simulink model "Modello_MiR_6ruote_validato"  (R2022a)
settings: Solver=VariableStepAuto  StartTime=0.0  StopTime=time_s(end,1)  RelTol=1e-3
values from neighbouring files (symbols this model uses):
  a = 0.250    (= 0.25)    [Modello_MiR_6ruote_validato_script.m]    (also in Modello_MiR_2ruote_script.m; Modello_MiR_6ruote_script.m; Modello_MiR_UR_script.m)
  a1 = 0.18265    [Modello_MiR_6ruote_validato_script.m]    (also in Modello_MiR_2ruote_script.m = deg2rad(5); Modello_MiR_6ruote_script.m = deg2rad(5); Modello_MiR_UR_script.m; UR_DHtable_e.m = 0)
  a2 = 0.40857    [Modello_MiR_6ruote_validato_script.m]    (also in Modello_MiR_2ruote_script.m = deg2rad(25); Modello_MiR_6ruote_script.m = deg2rad(25); Modello_MiR_UR_script.m; UR_DHtable_e.m = 612)
  Att_C1 = 0.01    [Modello_MiR_6ruote_validato_script.m]    (also in Modello_MiR_UR_script.m)
  Att_C2 = 0.01    [Modello_MiR_6ruote_validato_script.m]    (also in Modello_MiR_UR_script.m)
  Att_C5 = 0.01    [Modello_MiR_6ruote_validato_script.m]    (also in Modello_MiR_UR_script.m)
  Att_C6 = 0.01    [Modello_MiR_6ruote_validato_script.m]    (also in Modello_MiR_UR_script.m)
  b = 0.1875    [Modello_MiR_6ruote_validato_script.m]    (also in Modello_MiR_2ruote_script.m; Modello_MiR_6ruote_script.m; Modello_MiR_UR_script.m)
  b_caster = 0.07    [Modello_MiR_6ruote_validato_script.m]    (also in Modello_MiR_2ruote_script.m; Modello_MiR_6ruote_script.m; Modello_MiR_UR_script.m)
  bd = 0.205    [Modello_MiR_6ruote_validato_script.m]    (also in Modello_MiR_2ruote_script.m; Modello_MiR_6ruote_script.m; Modello_MiR_UR_script.m)
  F23fun = @(u) (mv*9.801/4)-(mv*h*u(5)+(mv*9.801/4)*(2*a-b_caster*(cos(u(1))+cos(u(2)))))/(4*a-b_caster*(cos(u(1))+cos(u(2)))+b_caster*(cos(u(3))+cos(u(4))))    [Modello_MiR_6ruote_validato_script.m]    (also in Modello_MiR_6ruote_script.m = @(u) (mv*9.801/4)-u(7))
  F43fun = @(u) (1/(2*bd))*(mv*u(6)*h+((mv*h*u(5)+(mv*9.801/4)*(2*a-b_caster*(cos(u(1))+cos(u(2)))))/(4*a-b_caster*(cos(u(1))+cos(u(2)))+b_caster*(cos(u(3))+cos(u(4)))))*(2*bd-b_caster*(sin(u(3))+sin(u(4))))+((mv*9.801/4)-(mv*h*u(5)+(mv*9.801/4)*(2*a-b_caster*(cos(u(1))+cos(u(2)))))/(4*a-b_caster*(cos(u(1))+cos(u(2)))+b_caster*(cos(u(3))+cos(u(4)))))*(2*bd-b_caster*(sin(u(1))+sin(u(2)))))    [Modello_MiR_6ruote_validato_script.m]    (also in Modello_MiR_6ruote_script.m = @(u) (1/(2*bd))*(mv*u(6)*h+u(7)*(2*bd-b_caster*(sin(u(3))+si)
  F63fun = @(u) (mv*h*u(5)+(mv*9.801/4)*(2*a-b_caster*(cos(u(1))+cos(u(2)))))/(4*a-b_caster*(cos(u(1))+cos(u(2)))+b_caster*(cos(u(3))+cos(u(4))))    [Modello_MiR_6ruote_validato_script.m]    (also in Modello_MiR_6ruote_script.m)
  f_c = 0.29564    [Modello_MiR_6ruote_validato_script.m]    (also in Modello_MiR_UR_script.m)
  f_d3 = 0.35846    [Modello_MiR_6ruote_validato_script.m]    (also in Modello_MiR_UR_script.m)
  f_d4 = 0.2333    [Modello_MiR_6ruote_validato_script.m]    (also in Modello_MiR_UR_script.m)
  fa_c = 0.27474    [Modello_MiR_6ruote_validato_script.m]    (also in Modello_MiR_UR_script.m)
  fa_d3 = 0.3694    [Modello_MiR_6ruote_validato_script.m]    (also in Modello_MiR_UR_script.m)
  fa_d4 = 0.28065    [Modello_MiR_6ruote_validato_script.m]    (also in Modello_MiR_UR_script.m)
  fm_fun = @(u) (u <= -am2 || u >= am2) * 0 + (u > -am2 && u <= -am1) * (- u* Mza/(am2 -am1) - Mza* am2/(am2 -am1)) +           + (u > -am1 && u <= am1) * (Mza * u / am1) + (u > am1 && u < am2) * (Mza * u /(am1 -am2) - Mza * am2 /(am1 - am2))    [Modello_MiR_6ruote_validato_script.m]    (also in Modello_MiR_6ruote_script.m = @(u) (u <= -am2 | u >= am2)*0 + (u > -am2 && u <= -am1)*(- u; Modello_MiR_UR_script.m)
  Icw_1 = 1/2 * mcw * rc^2    (= 0.002004225735)    [Modello_MiR_6ruote_validato_script.m]    (also in Modello_MiR_2ruote_script.m; Modello_MiR_6ruote_script.m; Modello_MiR_UR_script.m)
  Icw_2 = 1/12 * mcw * ec^2 + 1/4 * mcw * rc^2    (= 0.00104098243873)    [Modello_MiR_6ruote_validato_script.m]    (also in Modello_MiR_2ruote_script.m; Modello_MiR_6ruote_script.m; Modello_MiR_UR_script.m)
  Idw_1 = 1/2 * mdw * rd^2    (= 0.00551836278784)    [Modello_MiR_6ruote_validato_script.m]    (also in Modello_MiR_2ruote_script.m; Transfer_Function_Gol_Gcl.m = Inertia_vect(jj,1); Modello_MiR_6ruote_script.m; Modello_MiR_UR_script.m)
  iMax = 20.7*1.1    (= 22.77)    [Modello_MiR_6ruote_validato_script.m]    (also in Modello_MiR_2ruote_script.m; Modello_MiR_6ruote_script.m; Modello_MiR_UR_script.m)
  Iv = mv * (l^2 + w^2)  / 12    (= 8.95033333333)    [Modello_MiR_6ruote_validato_script.m]    (also in Modello_MiR_2ruote_script.m = 6.75343333333; Modello_MiR_6ruote_script.m = 6.75343333333; Modello_MiR_UR_script.m = 6.75343333333)
  Kc = 0.15    [Modello_MiR_6ruote_validato_script.m]    (also in Modello_MiR_2ruote_script.m; Modello_MiR_6ruote_script.m; Modello_MiR_UR_script.m)
  Ki_i = 1    [Modello_MiR_6ruote_validato_script.m]    (also in Modello_MiR_2ruote_script.m; Modello_MiR_6ruote_script.m; Modello_MiR_UR_script.m)
  Ki_v = 1    [Modello_MiR_6ruote_validato_script.m]    (also in Modello_MiR_2ruote_script.m; Modello_MiR_6ruote_script.m; Modello_MiR_UR_script.m)
  kk = 0.00005    (= 5e-05)    [Modello_MiR_6ruote_validato_script.m]    (also in Modello_MiR_2ruote_script.m; Modello_MiR_6ruote_script.m; Modello_MiR_UR_script.m)
  Kp_i = 5    [Modello_MiR_6ruote_validato_script.m]    (also in Modello_MiR_2ruote_script.m; Modello_MiR_6ruote_script.m; Modello_MiR_UR_script.m)
  Kp_v = 5    [Modello_MiR_6ruote_validato_script.m]    (also in Modello_MiR_2ruote_script.m; Modello_MiR_6ruote_script.m; Modello_MiR_UR_script.m)
  kv = 1.5e-6    (= 1.5e-06)    [Modello_MiR_6ruote_validato_script.m]    (also in Modello_MiR_2ruote_script.m; Modello_MiR_6ruote_script.m; Modello_MiR_UR_script.m)
  L = R * tauE    (= 0.00181134822805)    [Modello_MiR_6ruote_validato_script.m]    (also in Modello_MiR_2ruote_script.m; Modello_MiR_6ruote_script.m; Modello_MiR_UR_script.m)
  mcw = rc^2 * pi * ec * rhopoliu + 1    (= 1.02616357632)    [Modello_MiR_6ruote_validato_script.m]    (also in Modello_MiR_2ruote_script.m; Modello_MiR_6ruote_script.m; Modello_MiR_UR_script.m)
  mv = 110    [Modello_MiR_6ruote_validato_script.m]    (also in Modello_MiR_2ruote_script.m = 83; Modello_MiR_6ruote_script.m = 83; Modello_MiR_UR_script.m = 83)
  Phi1_start = psi_mir(1,1)    [Modello_MiR_6ruote_validato_script.m]    (also in Modello_MiR_UR_script.m)
  Phi2_start = psi_mir(1,1)    [Modello_MiR_6ruote_validato_script.m]    (also in Modello_MiR_UR_script.m)
  Phi5_start = psi_mir(1,1)    [Modello_MiR_6ruote_validato_script.m]    (also in Modello_MiR_UR_script.m)
  Phi6_start = psi_mir(1,1)    [Modello_MiR_6ruote_validato_script.m]    (also in Modello_MiR_UR_script.m)
  Psi_start = psi_mir(1,1)    [Modello_MiR_6ruote_validato_script.m]    (also in Modello_MiR_6ruote_script.m = 1.57079632679; Modello_MiR_UR_script.m)
  R = velMax * TorqueMax / (iMax)^2    (= 1.81134822805)    [Modello_MiR_6ruote_validato_script.m]    (also in Modello_MiR_2ruote_script.m; Modello_MiR_6ruote_script.m; Modello_MiR_UR_script.m)
  rap_rid = 10.167    [Modello_MiR_6ruote_validato_script.m]    (also in Modello_MiR_2ruote_script.m; Modello_MiR_6ruote_script.m; Modello_MiR_UR_script.m)
  rc = 0.125/2    (= 0.0625)    [Modello_MiR_6ruote_validato_script.m]    (also in Modello_MiR_2ruote_script.m; Modello_MiR_6ruote_script.m; Modello_MiR_UR_script.m)
  rd = 0.1    [Modello_MiR_6ruote_validato_script.m]    (also in Modello_MiR_2ruote_script.m; Modello_MiR_6ruote_script.m; Modello_MiR_UR_script.m)
  s1 = 0.18987    [Modello_MiR_6ruote_validato_script.m]    (also in Modello_MiR_2ruote_script.m = 0.2; Modello_MiR_6ruote_script.m = 0.2; Modello_MiR_UR_script.m)
  s2 = 0.99533    [Modello_MiR_6ruote_validato_script.m]    (also in Modello_MiR_2ruote_script.m = 0.8; Modello_MiR_6ruote_script.m = 0.8; Modello_MiR_UR_script.m)
  Sx = spline(x ,fl_fun(x),zx)    [Modello_MiR_6ruote_script.m]
  Sy = spline(x ,ft_fun(x),zy)    [Modello_MiR_6ruote_script.m]
  VaMax = Kc * velMax    (= 41.2443991527)    [Modello_MiR_6ruote_validato_script.m]    (also in Modello_MiR_2ruote_script.m; Modello_MiR_6ruote_script.m; Modello_MiR_UR_script.m)
  X_start = traj(1,1)    [Modello_MiR_6ruote_validato_script.m]    (also in Modello_MiR_2ruote_script.m = input('Inserire coordinata x iniziale'); Modello_MiR_6ruote_script.m = input('Inserire coordinata x iniziale'); Modello_MiR_UR_script.m)
  Y_start = traj(1,2)    [Modello_MiR_6ruote_validato_script.m]    (also in Modello_MiR_2ruote_script.m = input('Inserire coordinata y iniziale'); Modello_MiR_6ruote_script.m = input('Inserire coordinata y iniziale'); Modello_MiR_UR_script.m)
undefined symbols (not defined in the file or in its folder): z
libraries: slpidlib x4
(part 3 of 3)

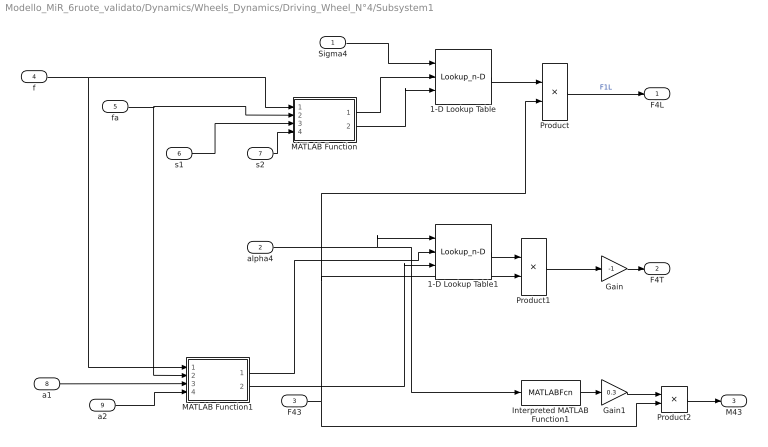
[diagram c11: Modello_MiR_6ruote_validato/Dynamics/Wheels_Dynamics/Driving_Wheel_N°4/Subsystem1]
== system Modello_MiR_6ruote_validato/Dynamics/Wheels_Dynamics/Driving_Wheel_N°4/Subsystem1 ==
  Sigma4 : Inport
  alpha4 : Inport  Port=2
  F43 : Inport  Port=3
  f : Inport  Port=4
  fa : Inport  Port=5
  s1 : Inport  Port=6
  s2 : Inport  Port=7
  a1 : Inport  Port=8
  a2 : Inport  Port=9
  1-D Lookup Table : Lookup_n-D  NumberOfTableDimensions=1  BreakpointsForDimension1Source=Input port  BreakpointsForDimension1=z  TableSource=Input port  Table=Sx  InternalRulePriority=Speed  RndMeth=Simplest
  1-D Lookup Table1 : Lookup_n-D  NumberOfTableDimensions=1  BreakpointsForDimension1Source=Input port  BreakpointsForDimension1=z  TableSource=Input port  Table=Sy  InternalRulePriority=Speed  RndMeth=Simplest
  Gain : Gain  Gain=-1
  Gain1 : Gain  Gain=0.3
  Interpreted MATLAB Function1 : MATLABFcn  MATLABFcn=fm_fun(u)
  MATLAB Function : MATLAB Function  TreatAsAtomicUnit=on
  MATLAB Function1 : MATLAB Function  TreatAsAtomicUnit=on
  Product : Product
  Product1 : Product
  Product2 : Product
  F4L : Outport
  F4T : Outport  Port=2
  M43 : Outport  Port=3
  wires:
  Gain/1 -> F4T/1
  Interpreted MATLAB Function1/1 -> Gain1/1
  F43/1 -> Product2/2, Product/2, Product1/2
  alpha4/1 -> Interpreted MATLAB Function1/1, 1-D Lookup Table1/1
  Product1/1 -> Gain/1
  Product/1 -> F4L/1  "F1L"
  1-D Lookup Table1/1 -> Product1/1
  1-D Lookup Table/1 -> Product/1
  Sigma4/1 -> 1-D Lookup Table/1
  s1/1 -> MATLAB Function/3(s1)
  MATLAB Function/2(z) -> 1-D Lookup Table/3
  MATLAB Function/1(Sx) -> 1-D Lookup Table/2
  s2/1 -> MATLAB Function/4(s2)
  a1/1 -> MATLAB Function1/3(a1)
  MATLAB Function1/1(Sy) -> 1-D Lookup Table1/2
  MATLAB Function1/2(z) -> 1-D Lookup Table1/3
  f/1 -> MATLAB Function1/1(f), MATLAB Function/1(f)
  a2/1 -> MATLAB Function1/4(a2)
  fa/1 -> MATLAB Function1/2(fa), MATLAB Function/2(fa)
  Product2/1 -> M43/1
  Gain1/1 -> Product2/1

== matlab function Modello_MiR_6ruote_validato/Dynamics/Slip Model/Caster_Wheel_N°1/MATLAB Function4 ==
function Fc_neg_out = fcn(v_wheel,Vx_DL)
x=v_wheel;
y=Vx_DL;
cccc=1e20;

Fc_neg=@(x,y) ((((x-y)/abs(y+((1/cccc)*(y==0))))*(((x-y)/abs(y+((1/cccc)*(y==0))))>=-1)+ (-1)*(((x-y)/abs(y+((1/cccc)*(y==0))))<-1))*(x*y>=0 && y>=0) + (((x-y)/abs(x+((1/cccc)*(x==0))))*(((x-y)/abs(x+((1/cccc)*(x==0))))>=-1))*(x*y>0 && y<0) + (x*y<0)*(x/abs(x+((1/cccc)*(x==0)))) )*(0.02<(x^2+y^2)) +(10*(x-y)*(10*(x-y)>-1) -1*(10*(x-y)<=-1))*(0.02>=(x^2+y^2)); 
Fc_neg_out = Fc_neg(x,y);

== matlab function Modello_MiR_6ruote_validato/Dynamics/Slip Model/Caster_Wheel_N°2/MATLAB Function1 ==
function Fc_pos_out = fcn(v_wheel,Vx_DL)
x=v_wheel;
y=Vx_DL;
cccc=1e20;

Fc_pos=@(x,y) ((((x-y)/abs(x+((1/cccc)*(x==0))))*(((x-y)/abs(x+((1/cccc)*(x==0))))<=1 )+ 1*(((x-y)/abs(x+((1/cccc)*(x==0))))>1))*(x*y>=0 && x>=0) + (((x-y)/abs(y+((1/cccc)*(y==0))))*(((x-y)/abs(y+((1/cccc)*(y==0))))<=1 ))*(x*y>0 && x<0)+ (x*y<0)*(x/abs(x+((1/cccc)*(x==0)))))*(0.02<(x^2+y^2)) + (10*(x-y)*(10*(x-y)<1) +1*(10*(x-y)>=1))*(0.02>=(x^2+y^2));

Fc_pos_out = Fc_pos(x,y);

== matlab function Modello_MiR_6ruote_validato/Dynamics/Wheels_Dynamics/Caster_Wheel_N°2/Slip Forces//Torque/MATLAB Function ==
function [Sx, z] = fcn(f, fa, s1, s2)

fla =  fa  ;
fl = f  ;
fl_fun = @(u) (u <= -s2).* (-fl) + (u > -s2 & u <= -s1).*(u*(fl - fla)/(s2 - s1) + s2*(fl - fla)/(s2 - s1) - fl) +...
              + (u > -s1 & u <= s1).*(u * fla / s1) + (u > s1 & u <= s2).* (u * (fla - fl)/(s1 - s2) - s2 * (fla - fl)/(s1 - s2) + fl) + ...
              + (u> s2) * fl;
% Interpolazione Cubica Attrito Longitudinale
nvet = 23 ; %specificare i numeri di nodi ( −1) della partizione
inferior = -1; % estremo inferiore intervallo
superi = 1 ; % estremo superiore intervallo
z = linspace(inferior,superi,10001); % definisco la griglia fine su cui valutare la spline

n = nvet ;
x = linspace(inferior, superi, n+1); % in questo esercizio definisco i nodi di interpolazione tra loro equispaziati
Sx = spline(x ,fl_fun(x),z) ; % valuto la spline cubica interpolante

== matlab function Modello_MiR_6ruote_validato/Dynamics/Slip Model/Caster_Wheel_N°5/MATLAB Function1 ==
function Fc_pos_out = fcn(v_wheel,Vx_DL)
x=v_wheel;
y=Vx_DL;
cccc=1e20;

Fc_pos=@(x,y) ((((x-y)/abs(x+((1/cccc)*(x==0))))*(((x-y)/abs(x+((1/cccc)*(x==0))))<=1 )+ 1*(((x-y)/abs(x+((1/cccc)*(x==0))))>1))*(x*y>=0 && x>=0) + (((x-y)/abs(y+((1/cccc)*(y==0))))*(((x-y)/abs(y+((1/cccc)*(y==0))))<=1 ))*(x*y>0 && x<0)+ (x*y<0)*(x/abs(x+((1/cccc)*(x==0)))))*(0.02<(x^2+y^2)) + (10*(x-y)*(10*(x-y)<1) +1*(10*(x-y)>=1))*(0.02>=(x^2+y^2));

Fc_pos_out = Fc_pos(x,y);

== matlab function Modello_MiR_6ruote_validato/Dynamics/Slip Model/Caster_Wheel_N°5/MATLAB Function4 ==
function Fc_neg_out = fcn(v_wheel,Vx_DL)
x=v_wheel;
y=Vx_DL;
cccc=1e20;

Fc_neg=@(x,y) ((((x-y)/abs(y+((1/cccc)*(y==0))))*(((x-y)/abs(y+((1/cccc)*(y==0))))>=-1)+ (-1)*(((x-y)/abs(y+((1/cccc)*(y==0))))<-1))*(x*y>=0 && y>=0) + (((x-y)/abs(x+((1/cccc)*(x==0))))*(((x-y)/abs(x+((1/cccc)*(x==0))))>=-1))*(x*y>0 && y<0) + (x*y<0)*(x/abs(x+((1/cccc)*(x==0)))) )*(0.02<(x^2+y^2)) +(10*(x-y)*(10*(x-y)>-1) -1*(10*(x-y)<=-1))*(0.02>=(x^2+y^2)); 
Fc_neg_out = Fc_neg(x,y);

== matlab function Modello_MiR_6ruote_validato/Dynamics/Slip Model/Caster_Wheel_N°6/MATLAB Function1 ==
function Fc_pos_out = fcn(v_wheel,Vx_DL)
x=v_wheel;
y=Vx_DL;
cccc=1e20;

Fc_pos=@(x,y) ((((x-y)/abs(x+((1/cccc)*(x==0))))*(((x-y)/abs(x+((1/cccc)*(x==0))))<=1 )+ 1*(((x-y)/abs(x+((1/cccc)*(x==0))))>1))*(x*y>=0 && x>=0) + (((x-y)/abs(y+((1/cccc)*(y==0))))*(((x-y)/abs(y+((1/cccc)*(y==0))))<=1 ))*(x*y>0 && x<0)+ (x*y<0)*(x/abs(x+((1/cccc)*(x==0)))))*(0.02<(x^2+y^2)) + (10*(x-y)*(10*(x-y)<1) +1*(10*(x-y)>=1))*(0.02>=(x^2+y^2));

Fc_pos_out = Fc_pos(x,y);

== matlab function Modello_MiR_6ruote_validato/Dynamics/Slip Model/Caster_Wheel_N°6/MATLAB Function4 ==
function Fc_neg_out = fcn(v_wheel,Vx_DL)
x=v_wheel;
y=Vx_DL;
cccc=1e20;

Fc_neg=@(x,y) ((((x-y)/abs(y+((1/cccc)*(y==0))))*(((x-y)/abs(y+((1/cccc)*(y==0))))>=-1)+ (-1)*(((x-y)/abs(y+((1/cccc)*(y==0))))<-1))*(x*y>=0 && y>=0) + (((x-y)/abs(x+((1/cccc)*(x==0))))*(((x-y)/abs(x+((1/cccc)*(x==0))))>=-1))*(x*y>0 && y<0) + (x*y<0)*(x/abs(x+((1/cccc)*(x==0)))) )*(0.02<(x^2+y^2)) +(10*(x-y)*(10*(x-y)>-1) -1*(10*(x-y)<=-1))*(0.02>=(x^2+y^2)); 
Fc_neg_out = Fc_neg(x,y);

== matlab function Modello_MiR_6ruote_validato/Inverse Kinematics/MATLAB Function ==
function Thetad_DR_SET = angvelR( xd_set, psid_set)
 bd = 0.2050;
 rd = 0.1;
Thetad_DR_SET = 1/rd * (xd_set + bd*psid_set);

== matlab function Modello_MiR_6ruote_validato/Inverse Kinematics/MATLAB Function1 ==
function Thetad_DL_SET = angvelL(xd_set,  psid_set)
 bd = 0.2050;
 rd = 0.1;
Thetad_DL_SET = 1/rd * (xd_set - bd*psid_set);

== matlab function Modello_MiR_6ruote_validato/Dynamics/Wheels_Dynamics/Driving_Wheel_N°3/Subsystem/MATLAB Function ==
function [Sx, z] = fcn(f, fa, s1, s2)

fla =  fa  ;
fl = f  ;
fl_fun = @(u) (u <= -s2).* (-fl) + (u > -s2 & u <= -s1).*(u*(fl - fla)/(s2 - s1) + s2*(fl - fla)/(s2 - s1) - fl) +...
              + (u > -s1 & u <= s1).*(u * fla / s1) + (u > s1 & u <= s2).* (u * (fla - fl)/(s1 - s2) - s2 * (fla - fl)/(s1 - s2) + fl) + ...
              + (u> s2) * fl;

% Interpolazione Cubica Attrito Longitudinale
nvet = 23 ; %specificare i numeri di nodi ( −1) della partizione
inferior = -1; % estremo inferiore intervallo
superi = 1 ; % estremo superiore intervallo
z = linspace(inferior,superi,10001); % definisco la griglia fine su cui valutare la spline

n = nvet ;
x = linspace(inferior, superi, n+1); % in questo esercizio definisco i nodi di interpolazione tra loro equispaziati
Sx = spline(x ,fl_fun(x),z) ; % valuto la spline cubica interpolante

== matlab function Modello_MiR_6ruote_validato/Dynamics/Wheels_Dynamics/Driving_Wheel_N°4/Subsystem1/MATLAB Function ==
function [Sx, z] = fcn(f, fa, s1, s2)

fla =  fa  ;
fl = f  ;
Fx = @(u) (u <= -s2).* (-fl) + (u > -s2 & u <= -s1).*(u*(fl - fla)/(s2 - s1) + s2*(fl - fla)/(s2 - s1) - fl) +...
          + (u > -s1 & u <= s1).*(u * fla / s1) + (u > s1 & u <= s2).* (u * (fla - fl)/(s1 - s2) - s2 * (fla - fl)/(s1 - s2) + fl) + ...
          + (u> s2) * fl;

% Interpolazione Cubica Attrito Longitudinale
nvet = 23 ; %specificare i numeri di nodi ( −1) della partizione
inferior = -1; % estremo inferiore intervallo
superi = 1 ; % estremo superiore intervallo
z = linspace(inferior,superi,10001); % definisco la griglia fine su cui valutare la spline

n = nvet ;
x = linspace(inferior, superi, n+1); % in questo esercizio definisco i nodi di interpolazione tra loro equispaziati
Sx = spline(x ,Fx(x),z) ; % valuto la spline cubica interpolante

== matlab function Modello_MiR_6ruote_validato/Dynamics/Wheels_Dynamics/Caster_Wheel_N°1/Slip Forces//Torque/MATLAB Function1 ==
function [Sy, z] = fcn(f, fa, a1, a2)

fta = 1200/2500/0.6 * fa;
ft = 1200/2500/0.6 * f;
ft_fun = @(u) (u <= -a2).*(-ft) + (u > -a2 & u <= -a1).* (u*(ft - fta)/(a2 - a1) + a2*(ft - fta)/(a2 - a1) - ft) +...
              + (u > -a1 & u <= a1).* (u * fta / a1) + (u > a1 & u <= a2).* (u * (fta - ft)/(a1 - a2) - a2 * (fta - ft)/(a1 - a2) + ft) + ...
              + (u > a2).* ft;

nvet = 20 ; %specificare i numeri di nodi ( −1) della partizione
inferior = -pi/2; % estremo inferiore intervallo
superi = pi/2 ; % estremo superiore intervallo
z = linspace(inferior,superi,10001); % definisco la griglia fine su cui valutare la spline

n = nvet ;
x = linspace(inferior, superi, n+1); % in questo esercizio definisco i nodi di interpolazione tra loro equispaziati
Sy = spline(x ,ft_fun(x),z) ; % valuto la spline cubica interpolante

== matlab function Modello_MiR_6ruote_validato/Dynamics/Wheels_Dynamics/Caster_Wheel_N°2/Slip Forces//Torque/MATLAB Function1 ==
function [Sy, z] = fcn(f, fa, a1, a2)

fta = 1200/2500/0.6 * fa;
ft = 1200/2500/0.6 * f;
ft_fun = @(u) (u <= -a2).*(-ft) + (u > -a2 & u <= -a1).* (u*(ft - fta)/(a2 - a1) + a2*(ft - fta)/(a2 - a1) - ft) +...
              + (u > -a1 & u <= a1).* (u * fta / a1) + (u > a1 & u <= a2).* (u * (fta - ft)/(a1 - a2) - a2 * (fta - ft)/(a1 - a2) + ft) + ...
              + (u > a2).* ft;

nvet = 20 ; %specificare i numeri di nodi ( −1) della partizione
inferior = -pi/2; % estremo inferiore intervallo
superi = pi/2 ; % estremo superiore intervallo
z = linspace(inferior,superi,10001); % definisco la griglia fine su cui valutare la spline

n = nvet ;
x = linspace(inferior, superi, n+1); % in questo esercizio definisco i nodi di interpolazione tra loro equispaziati
Sy = spline(x ,ft_fun(x),z) ; % valuto la spline cubica interpolante

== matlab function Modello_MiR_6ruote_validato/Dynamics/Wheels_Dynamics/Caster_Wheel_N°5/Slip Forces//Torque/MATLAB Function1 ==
function [Sy, z] = fcn(f, fa, a1, a2)

fta = 1200/2500/0.6 * fa;
ft = 1200/2500/0.6 * f;
ft_fun = @(u) (u <= -a2).*(-ft) + (u > -a2 & u <= -a1).* (u*(ft - fta)/(a2 - a1) + a2*(ft - fta)/(a2 - a1) - ft) +...
              + (u > -a1 & u <= a1).* (u * fta / a1) + (u > a1 & u <= a2).* (u * (fta - ft)/(a1 - a2) - a2 * (fta - ft)/(a1 - a2) + ft) + ...
              + (u > a2).* ft;

nvet = 20 ; %specificare i numeri di nodi ( −1) della partizione
inferior = -pi/2; % estremo inferiore intervallo
superi = pi/2 ; % estremo superiore intervallo
z = linspace(inferior,superi,10001); % definisco la griglia fine su cui valutare la spline

n = nvet ;
x = linspace(inferior, superi, n+1); % in questo esercizio definisco i nodi di interpolazione tra loro equispaziati
Sy = spline(x ,ft_fun(x),z) ; % valuto la spline cubica interpolante

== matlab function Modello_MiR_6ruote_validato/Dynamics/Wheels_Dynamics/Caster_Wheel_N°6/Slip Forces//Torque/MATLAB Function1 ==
function [Sy, z] = fcn(f, fa, a1, a2)

fta = 1200/2500/0.6 * fa;
ft = 1200/2500/0.6 * f;
ft_fun = @(u) (u <= -a2).*(-ft) + (u > -a2 & u <= -a1).* (u*(ft - fta)/(a2 - a1) + a2*(ft - fta)/(a2 - a1) - ft) +...
              + (u > -a1 & u <= a1).* (u * fta / a1) + (u > a1 & u <= a2).* (u * (fta - ft)/(a1 - a2) - a2 * (fta - ft)/(a1 - a2) + ft) + ...
              + (u > a2).* ft;

nvet = 20 ; %specificare i numeri di nodi ( −1) della partizione
inferior = -pi/2; % estremo inferiore intervallo
superi = pi/2 ; % estremo superiore intervallo
z = linspace(inferior,superi,10001); % definisco la griglia fine su cui valutare la spline

n = nvet ;
x = linspace(inferior, superi, n+1); % in questo esercizio definisco i nodi di interpolazione tra loro equispaziati
Sy = spline(x ,ft_fun(x),z) ; % valuto la spline cubica interpolante

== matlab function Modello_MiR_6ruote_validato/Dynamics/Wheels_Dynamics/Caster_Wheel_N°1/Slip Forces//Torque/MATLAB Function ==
function [Sx, z] = fcn(f, fa, s1, s2)

fla =  fa  ;
fl = f  ;
fl_fun = @(u) (u <= -s2).* (-fl) + (u > -s2 & u <= -s1).*(u*(fl - fla)/(s2 - s1) + s2*(fl - fla)/(s2 - s1) - fl) +...
              + (u > -s1 & u <= s1).*(u * fla / s1) + (u > s1 & u <= s2).* (u * (fla - fl)/(s1 - s2) - s2 * (fla - fl)/(s1 - s2) + fl) + ...
              + (u> s2) * fl;

% Interpolazione Cubica Attrito Longitudinale
nvet = 23 ; %specificare i numeri di nodi ( −1) della partizione
inferior = -1; % estremo inferiore intervallo
superi = 1 ; % estremo superiore intervallo
z = linspace(inferior,superi,10001); % definisco la griglia fine su cui valutare la spline


n = nvet ;
x = linspace(inferior, superi, n+1); % in questo esercizio definisco i nodi di interpolazione tra loro equispaziati
Sx = spline(x ,fl_fun(x),z) ; % valuto la spline cubica interpolante

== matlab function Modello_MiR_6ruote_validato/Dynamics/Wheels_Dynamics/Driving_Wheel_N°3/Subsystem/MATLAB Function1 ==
function [Sy, z] = fcn(f, fa, a1, a2)

fta = 1200/2500/0.6 * fa;
ft = 1200/2500/0.6 * f;
ft_fun = @(u) (u <= -a2).*(-ft) + (u > -a2 & u <= -a1).* (u*(ft - fta)/(a2 - a1) + a2*(ft - fta)/(a2 - a1) - ft) +...
              + (u > -a1 & u <= a1).* (u * fta / a1) + (u > a1 & u <= a2).* (u * (fta - ft)/(a1 - a2) - a2 * (fta - ft)/(a1 - a2) + ft) + ...
              + (u > a2).* ft;

nvet = 20 ; %specificare i numeri di nodi ( −1) della partizione
inferior = -pi/2; % estremo inferiore intervallo
superi = pi/2 ; % estremo superiore intervallo
z = linspace(inferior,superi,10001); % definisco la griglia fine su cui valutare la spline

n = nvet ;
x = linspace(inferior, superi, n+1); % in questo esercizio definisco i nodi di interpolazione tra loro equispaziati
Sy = spline(x ,ft_fun(x),z) ; % valuto la spline cubica interpolante

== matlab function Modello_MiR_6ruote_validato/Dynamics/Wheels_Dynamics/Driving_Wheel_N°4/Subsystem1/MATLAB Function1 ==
function [Sy, z] = fcn(f, fa, a1, a2)

fta = 1200/2500/0.6 * fa;
ft = 1200/2500/0.6 * f;
ft_fun = @(u) (u <= -a2).*(-ft) + (u > -a2 & u <= -a1).* (u*(ft - fta)/(a2 - a1) + a2*(ft - fta)/(a2 - a1) - ft) +...
              + (u > -a1 & u <= a1).* (u * fta / a1) + (u > a1 & u <= a2).* (u * (fta - ft)/(a1 - a2) - a2 * (fta - ft)/(a1 - a2) + ft) + ...
              + (u > a2).* ft;

nvet = 20 ; %specificare i numeri di nodi ( −1) della partizione
inferior = -pi/2; % estremo inferiore intervallo
superi = pi/2 ; % estremo superiore intervallo
z = linspace(inferior,superi,10001); % definisco la griglia fine su cui valutare la spline

n = nvet ;
x = linspace(inferior, superi, n+1); % in questo esercizio definisco i nodi di interpolazione tra loro equispaziati
Sy = spline(x ,ft_fun(x),z) ; % valuto la spline cubica interpolante

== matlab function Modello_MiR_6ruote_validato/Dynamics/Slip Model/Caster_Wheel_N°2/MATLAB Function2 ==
function Fc_neg_out = fcn(v_wheel,Vx_DL)
x=v_wheel;
y=Vx_DL;
cccc=1e20;

Fc_neg=@(x,y) ((((x-y)/abs(y+((1/cccc)*(y==0))))*(((x-y)/abs(y+((1/cccc)*(y==0))))>=-1)+ (-1)*(((x-y)/abs(y+((1/cccc)*(y==0))))<-1))*(x*y>=0 && y>=0) + (((x-y)/abs(x+((1/cccc)*(x==0))))*(((x-y)/abs(x+((1/cccc)*(x==0))))>=-1))*(x*y>0 && y<0) + (x*y<0)*(x/abs(x+((1/cccc)*(x==0)))) )*(0.02<(x^2+y^2)) +(10*(x-y)*(10*(x-y)>-1) -1*(10*(x-y)<=-1))*(0.02>=(x^2+y^2)); 
Fc_neg_out = Fc_neg(x,y);

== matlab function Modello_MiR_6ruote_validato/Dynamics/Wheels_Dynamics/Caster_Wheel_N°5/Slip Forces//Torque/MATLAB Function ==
function [Sx, z] = fcn(f, fa, s1, s2)

fla =  fa  ;
fl = f  ;
fl_fun = @(u) (u <= -s2).* (-fl) + (u > -s2 & u <= -s1).*(u*(fl - fla)/(s2 - s1) + s2*(fl - fla)/(s2 - s1) - fl) +...
          + (u > -s1 & u <= s1).*(u * fla / s1) + (u > s1 & u <= s2).* (u * (fla - fl)/(s1 - s2) - s2 * (fla - fl)/(s1 - s2) + fl) + ...
          + (u> s2) * fl;

% Interpolazione Cubica Attrito Longitudinale
nvet = 23 ; %specificare i numeri di nodi ( −1) della partizione
inferior = -1; % estremo inferiore intervallo
superi = 1 ; % estremo superiore intervallo
z = linspace(inferior,superi,10001); % definisco la griglia fine su cui valutare la spline

n = nvet ;
x = linspace(inferior, superi, n+1); % in questo esercizio definisco i nodi di interpolazione tra loro equispaziati
Sx = spline(x ,fl_fun(x),z) ; % valuto la spline cubica interpolante

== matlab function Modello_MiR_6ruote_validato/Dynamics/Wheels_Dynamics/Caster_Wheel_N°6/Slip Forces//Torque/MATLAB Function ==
function [Sx, z] = fcn(f, fa, s1, s2)

fla =  fa  ;
fl = f  ;
fl_fun = @(u) (u <= -s2).* (-fl) + (u > -s2 & u <= -s1).*(u*(fl - fla)/(s2 - s1) + s2*(fl - fla)/(s2 - s1) - fl) +...
              + (u > -s1 & u <= s1).*(u * fla / s1) + (u > s1 & u <= s2).* (u * (fla - fl)/(s1 - s2) - s2 * (fla - fl)/(s1 - s2) + fl) + ...
              + (u> s2) * fl;

% Interpolazione Cubica Attrito Longitudinale
nvet = 23 ; %specificare i numeri di nodi ( −1) della partizione
inferior = -1; % estremo inferiore intervallo
superi = 1 ; % estremo superiore intervallo
z = linspace(inferior,superi,10001); % definisco la griglia fine su cui valutare la spline

n = nvet ;
x = linspace(inferior, superi, n+1); % in questo esercizio definisco i nodi di interpolazione tra loro equispaziati
Sx = spline(x ,fl_fun(x),z) ; % valuto la spline cubica interpolante

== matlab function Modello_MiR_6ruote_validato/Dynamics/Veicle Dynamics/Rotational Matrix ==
function [Fx_generalized, Fy_generalized] = fcn(FL,FT,Delta)
Fx_generalized=ones(6,1);
Fy_generalized=ones(6,1);

Fx_generalized(1,1)=FL(1)*cos(Delta(1))-FT(1)*sin(Delta(1));
Fy_generalized(1,1)=FT(1)*cos(Delta(1))+FL(1)*sin(Delta(1));
Fx_generalized(2,1)=FL(2)*cos(Delta(2))-FT(2)*sin(Delta(2));
Fy_generalized(2,1)=FT(2)*cos(Delta(2))+FL(2)*sin(Delta(2));
Fx_generalized(3,1)=FL(3);
Fy_generalized(3,1)=FT(3);
Fx_generalized(4,1)=FL(4);
Fy_generalized(4,1)=FT(4);
Fx_generalized(5,1)=FL(5)*cos(Delta(3))-FT(5)*sin(Delta(3));
Fy_generalized(5,1)=FT(5)*cos(Delta(3))+FL(5)*sin(Delta(3));
Fx_generalized(6,1)=FL(6)*cos(Delta(4))-FT(6)*sin(Delta(4));
Fy_generalized(6,1)=FT(6)*cos(Delta(4))+FL(6)*sin(Delta(4));

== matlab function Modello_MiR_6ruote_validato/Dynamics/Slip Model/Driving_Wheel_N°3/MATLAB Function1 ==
function Fc_pos_out = fcn(v_wheel,Vx_DL)

x=v_wheel;
y=Vx_DL;
cccc=1e20;

Fc_pos=@(x,y) ((((x-y)/abs(x+((1/cccc)*(x==0))))*(((x-y)/abs(x+((1/cccc)*(x==0))))<=1 )+ 1*(((x-y)/abs(x+((1/cccc)*(x==0))))>1))*(x*y>=0 && x>=0) + (((x-y)/abs(y+((1/cccc)*(y==0))))*(((x-y)/abs(y+((1/cccc)*(y==0))))<=1 ))*(x*y>0 && x<0)+ (x*y<0)*(x/abs(x+((1/cccc)*(x==0)))))*(0.02<(x^2+y^2)) + (10*(x-y)*(10*(x-y)<1) +1*(10*(x-y)>=1))*(0.02>=(x^2+y^2));

Fc_pos_out = Fc_pos(x,y);

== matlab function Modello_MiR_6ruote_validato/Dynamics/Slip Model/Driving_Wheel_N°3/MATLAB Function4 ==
function Fc_neg_out = fcn(v_wheel,Vx_DL)

x=v_wheel;
y=Vx_DL;
cccc=1e20;

Fc_neg=@(x,y) ((((x-y)/abs(y+((1/cccc)*(y==0))))*(((x-y)/abs(y+((1/cccc)*(y==0))))>=-1)+ (-1)*(((x-y)/abs(y+((1/cccc)*(y==0))))<-1))*(x*y>=0 && y>=0) + (((x-y)/abs(x+((1/cccc)*(x==0))))*(((x-y)/abs(x+((1/cccc)*(x==0))))>=-1))*(x*y>0 && y<0) + (x*y<0)*(x/abs(x+((1/cccc)*(x==0)))) )*(0.02<(x^2+y^2)) +(10*(x-y)*(10*(x-y)>-1) -1*(10*(x-y)<=-1))*(0.02>=(x^2+y^2)); 
Fc_neg_out = Fc_neg(x,y);

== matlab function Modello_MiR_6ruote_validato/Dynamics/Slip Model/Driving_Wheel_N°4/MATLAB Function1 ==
function Fc_pos_out = fcn(v_wheel,Vx_DL)
x=v_wheel;
y=Vx_DL;
cccc=1e20;

Fc_pos=@(x,y) ((((x-y)/abs(x+((1/cccc)*(x==0))))*(((x-y)/abs(x+((1/cccc)*(x==0))))<=1 )+ 1*(((x-y)/abs(x+((1/cccc)*(x==0))))>1))*(x*y>=0 && x>=0) + (((x-y)/abs(y+((1/cccc)*(y==0))))*(((x-y)/abs(y+((1/cccc)*(y==0))))<=1 ))*(x*y>0 && x<0)+ (x*y<0)*(x/abs(x+((1/cccc)*(x==0)))))*(0.02<(x^2+y^2)) + (10*(x-y)*(10*(x-y)<1) +1*(10*(x-y)>=1))*(0.02>=(x^2+y^2));

Fc_pos_out = Fc_pos(x,y);

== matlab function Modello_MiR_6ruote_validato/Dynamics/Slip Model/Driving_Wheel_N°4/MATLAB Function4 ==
function Fc_neg_out = fcn(v_wheel,Vx_DL)
x=v_wheel;
y=Vx_DL;
cccc=1e20;

Fc_neg=@(x,y) ((((x-y)/abs(y+((1/cccc)*(y==0))))*(((x-y)/abs(y+((1/cccc)*(y==0))))>=-1)+ (-1)*(((x-y)/abs(y+((1/cccc)*(y==0))))<-1))*(x*y>=0 && y>=0) + (((x-y)/abs(x+((1/cccc)*(x==0))))*(((x-y)/abs(x+((1/cccc)*(x==0))))>=-1))*(x*y>0 && y<0) + (x*y<0)*(x/abs(x+((1/cccc)*(x==0)))) )*(0.02<(x^2+y^2)) +(10*(x-y)*(10*(x-y)>-1) -1*(10*(x-y)<=-1))*(0.02>=(x^2+y^2)); 
Fc_neg_out = Fc_neg(x,y);

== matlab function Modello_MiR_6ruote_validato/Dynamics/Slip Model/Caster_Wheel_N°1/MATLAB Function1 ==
function Fc_pos_out = fcn(v_wheel,Vx_DL)
x=v_wheel;
y=Vx_DL;
cccc=1e20;

Fc_pos=@(x,y) ((((x-y)/abs(x+((1/cccc)*(x==0))))*(((x-y)/abs(x+((1/cccc)*(x==0))))<=1 )+ 1*(((x-y)/abs(x+((1/cccc)*(x==0))))>1))*(x*y>=0 && x>=0) + (((x-y)/abs(y+((1/cccc)*(y==0))))*(((x-y)/abs(y+((1/cccc)*(y==0))))<=1 ))*(x*y>0 && x<0)+ (x*y<0)*(x/abs(x+((1/cccc)*(x==0)))))*(0.02<(x^2+y^2)) + (10*(x-y)*(10*(x-y)<1) +1*(10*(x-y)>=1))*(0.02>=(x^2+y^2));

Fc_pos_out = Fc_pos(x,y);
